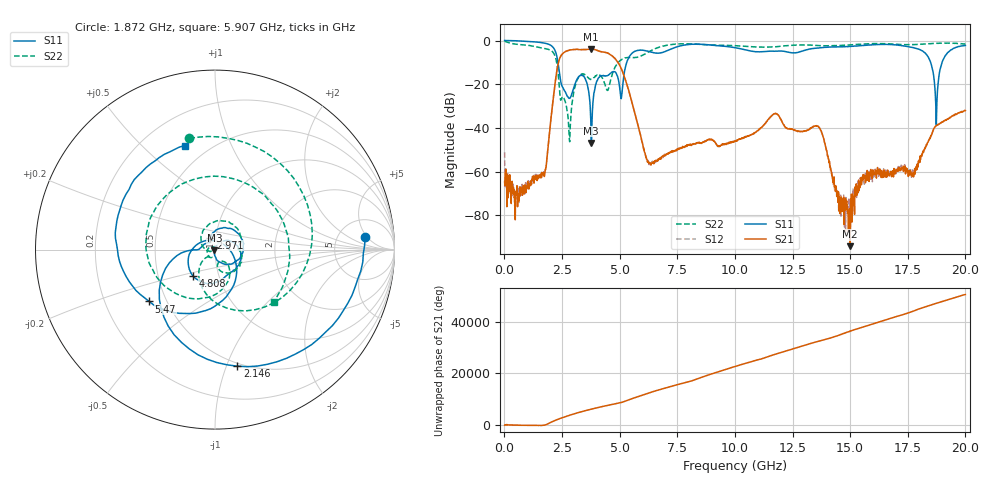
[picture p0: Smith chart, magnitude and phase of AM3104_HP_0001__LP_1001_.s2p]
!Created with skrf (http://scikit-rf.org).
# Hz S RI R 50.0
!freq ReS11 ImS11 ReS21 ImS21 ReS12 ImS12 ReS22 ImS22
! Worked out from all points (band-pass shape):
!   1601 points, 10 MHz to 20 GHz, reference 50 ohm
!   highest |S21| = -3.86 dB at 3.746 GHz (marker M1); lowest = -94.1 dB at 14.99 GHz (marker M2)
!   |S21| within 3 dB of the highest: 2.462 GHz to 4.652 GHz (2.189 GHz wide, 61.6 % of centre)
!   lowest |S11| = -46.8 dB at 3.771 GHz (marker M3), VSWR 1.01, Z = 49.7 - j0.332 ohm
!   |S11| at or under -10 dB: 2.324 GHz to 5.308 GHz (2.984 GHz wide, 78.2 % of centre); 18.49 GHz to 18.99 GHz (497 MHz wide, 2.65 % of centre)
!   |S22| runs from -46.3 to -0.2 dB; largest |S21 - S12| = 0.0058
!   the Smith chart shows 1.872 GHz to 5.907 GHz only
!   S11 on the Smith chart (normalised r, x): 1.872 GHz: 9, +5; 2.146 GHz: 0.47, -1.09; 2.971 GHz: 0.94, +0.13; 4.808 GHz: 0.75, -0.22; 5.47 GHz: 0.40, -0.30; 5.907 GHz: 0.37, +0.68
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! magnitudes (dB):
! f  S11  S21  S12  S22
! 10 MHz  0.0  -64.5  -51.1  -0.2
! 534.7 MHz  -0.1  -68.6  -69.3  -1.7
! 1.872 GHz  -1.5  -50.9  -50.9  -3.9
! 2.146 GHz  -3.6  -24.3  -24.3  -5.9
! 2.784 GHz  -26.2  -4.5  -4.5  -38.3
! 2.971 GHz  -22.9  -4.2  -4.2  -25.9
! 3.346 GHz  -15.8  -4.2  -4.2  -15.4
! 3.746 GHz  -35.7  -3.9  -3.9  -17.8
! 3.771 GHz  -46.8  -3.9  -3.9  -17.8
! 4.808 GHz  -14.4  -8.3  -8.3  -12.0
! 5.07 GHz  -26.6  -12.8  -12.8  -8.8
! 5.47 GHz  -6.6  -25.7  -25.7  -7.8
! 5.907 GHz  -4.4  -43.2  -43.4  -7.1
! 6.682 GHz  -5.8  -54.3  -54.5  -3.2
! 10.01 GHz  -3.3  -45.8  -45.9  -2.4
! 13.34 GHz  -3.7  -39.8  -39.8  -2.2
! 14.99 GHz  -2.7  -94.1  -73.4  -2.0
! 16.68 GHz  -1.8  -61.3  -59.9  -1.5
! 18.26 GHz  -5.8  -49.1  -49.4  -1.6
! 18.74 GHz  -38.5  -38.8  -39.1  -1.3
! 19.11 GHz  -7.2  -36.6  -36.6  -1.2
! 20 GHz  -2.3  -32.0  -32.0  -1.6
